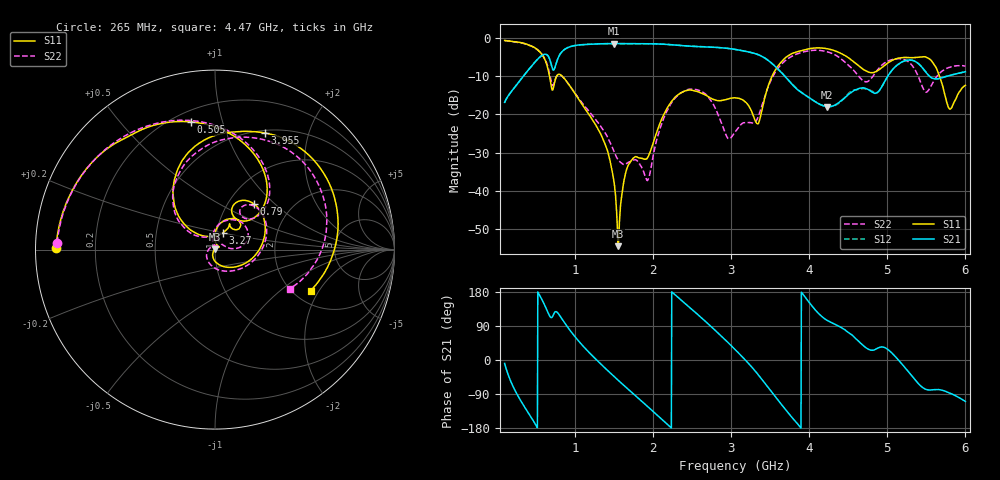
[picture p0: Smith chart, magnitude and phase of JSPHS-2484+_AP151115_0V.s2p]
!Mini-Circuits Laboratory
!S-Parameters
!Run/Lot/Date Code:MF33450/NA/1551
!Fixture/SN/Due: 90-4-20-21/70546/03/17/16
!Connection:PORT<IN> - pin<1>; PORT<OUT> - pin<7>;PORT<BIAS> - pin<4>;
!Tested With:PORT EXTENTION
!Network Analyzer:AG E5071C/74883/05/12/16
!Created: 01-07-2016 at 14:06:11
!MODEL: JSPHS-2484+
!S/N: V=0V
# MHZ S DB R 50
!Frequency  S11 dB  S11 DEG  S21 dB  S21 DEG  S12 dB  S12 DEG  S22 dB  S22 DEG
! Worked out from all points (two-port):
!   1181 points, 100 MHz to 6 GHz, reference 50 ohm
!   highest |S21| = -1.46 dB at 1.5 GHz (marker M1); lowest = -18.0 dB at 4.23 GHz (marker M2)
!   |S21| within 3 dB of the highest: 587.5 MHz to 646.4 MHz (58.95 MHz wide, 9.56 % of centre); 803.8 MHz to 3.358 GHz (2.555 GHz wide, 123 % of centre)
!   lowest |S11| = -54.5 dB at 1.555 GHz (marker M3), VSWR 1.00, Z = 49.8 + j0.113 ohm
!   |S11| at or under -10 dB: 674.8 MHz to 765.6 MHz (90.8 MHz wide, 12.6 % of centre); 838.6 MHz to 3.525 GHz (2.686 GHz wide, 123 % of centre); 5.668 GHz to end of sweep
!   |S22| runs from -37.3 to -0.7 dB; largest |S21 - S12| = 0.01
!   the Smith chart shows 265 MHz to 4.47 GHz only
!   S11 on the Smith chart (normalised r, x): 265 MHz: 0.06, +0.01; 505 MHz: 0.27, +0.80; 790 MHz: 1.31, +0.75; 3.27 GHz: 1.08, +0.21; 3.955 GHz: 0.53, +1.38; 4.47 GHz: 2.44, -1.70
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100  -0.64 -98.5  -16.86 -9.1  -16.86 -9.1  -0.67 -98.8
265  -1.05 179.3  -11.95 -92.6  -11.95 -92.5  -1.11 177.5
505  -2.81 100.5  -5.93 -173.3  -5.93 -173.3  -2.83 97.9
790  -9.51 49.4  -5.00 121.9  -5.00 121.9  -9.60 43.0
1085  -17.14 -45.2  -1.76 41.2  -1.76 41.2  -16.79 -56.1
1500  -37.56 -132.1  -1.46 -43.3  -1.46 -43.3  -29.62 173.4
1555  -54.50 142.9  -1.46 -53.6  -1.46 -53.7  -31.97 141.7
1680  -33.44 38.3  -1.48 -76.8  -1.47 -76.8  -32.60 67.1
1930  -31.41 63.4  -1.50 -122.6  -1.50 -122.6  -37.32 60.4
2070  -23.38 91.3  -1.56 -148.5  -1.56 -148.5  -25.02 104.6
2630  -14.53 41.9  -2.26 109.6  -2.26 109.5  -14.08 20.8
3050  -15.66 60.5  -2.98 27.9  -2.98 27.9  -24.65 74.1
3270  -19.58 64.3  -3.86 -19.8  -3.88 -19.9  -22.24 104.6
3955  -3.01 66.9  -15.03 164.1  -15.02 164.1  -3.51 67.2
4035  -2.70 54.9  -16.15 142.7  -16.14 142.7  -3.25 54.3
4230  -2.80 22.6  -18.03 104.7  -17.97 104.3  -3.61 20.8
4470  -4.73 -23.5  -15.39 77.4  -15.25 79.0  -6.52 -27.8
4765  -8.96 -107.8  -13.64 27.6  -13.54 28.8  -11.16 -153.8
5020  -6.35 136.3  -9.56 25.8  -9.56 25.7  -5.93 105.2
5495  -5.00 23.0  -8.97 -77.6  -8.96 -77.6  -14.16 58.9
5795  -18.55 1.3  -9.81 -86.6  -9.83 -86.6  -7.69 70.6
6000  -12.38 24.4  -8.83 -109.4  -8.84 -109.5  -7.38 54.2
